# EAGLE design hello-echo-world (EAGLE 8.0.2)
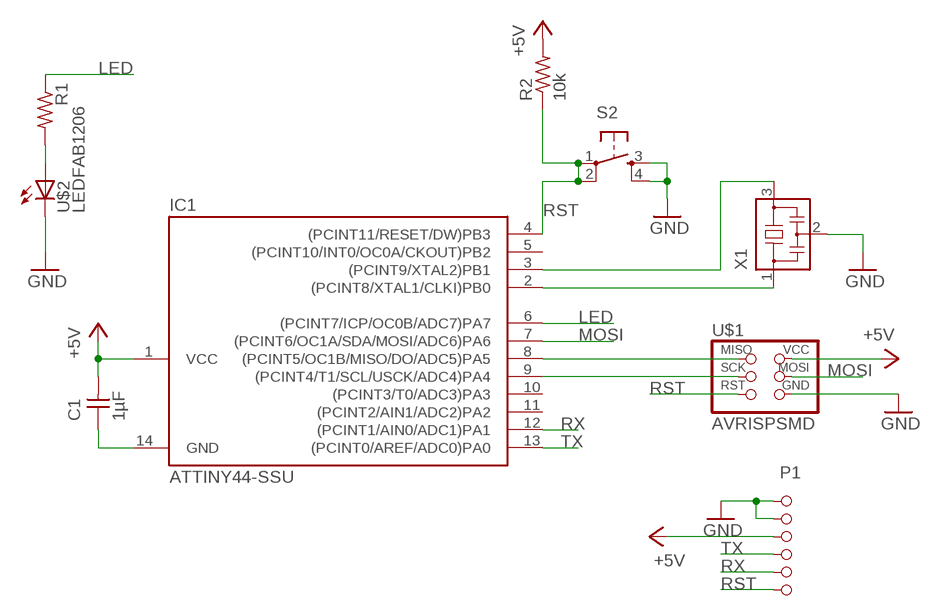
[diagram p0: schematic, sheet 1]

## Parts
C1  1µF  CAP-UNPOLARIZEDFAB  [C1206FAB]
IC1  ATTINY44-SSU  [SOIC14]
P1  SMD-6  [SMD-6]
R1  RES-US1206FAB  [R1206FAB]
R2  10k  RES-US1206FAB  [R1206FAB]
S2  6MM_SWITCH6MM_SWITCH  [6MM_SWITCH]
U$1  AVRISPSMD  [2X03SMD]
U$2  LEDFAB1206  [LED1206FAB]
X1  RESONATOR-PBRC  [PBRC]

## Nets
+5V: C1.2 IC1.1(VCC) P1.P$3 R2.2 U$1.2(VCC)
GND: C1.1 IC1.14(GND) P1.P$1 P1.P$2 S2.3(S) S2.4(S1) U$1.6(GND) U$2.2(C) X1.2
LED: IC1.6((PCINT7/ICP/OC0B/ADC7)PA7) R1.1
MOSI: IC1.7((PCINT6/OC1A/SDA/MOSI/ADC6)PA6) U$1.4(MOSI)
N$3: IC1.2((PCINT8/XTAL1/CLKI)PB0) X1.1
N$4: IC1.3((PCINT9/XTAL2)PB1) X1.3
N$5: IC1.8((PCINT5/OC1B/MISO/DO/ADC5)PA5) U$1.1(MISO)
N$6: IC1.9((PCINT4/T1/SCL/USCK/ADC4)PA4) U$1.3(SCK)
N$7: R1.2 U$2.1(A)
RST: IC1.4((PCINT11/RESET/DW)PB3) P1.P$6 R2.1 S2.1(P) S2.2(P1) U$1.5(RST)
RX: IC1.12((PCINT1/AIN0/ADC1)PA1) P1.P$5
TX: IC1.13((PCINT0/AREF/ADC0)PA0) P1.P$4
Unconnected: IC1.5((PCINT10/INT0/OC0A/CKOUT)PB2) IC1.10((PCINT3/T0/ADC3)PA3) IC1.11((PCINT2/AIN1/ADC2)PA2)

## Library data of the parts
C1 = fab:CAP-UNPOLARIZED
IC1 = fab:ATTINY44
P1 = PinHeader:SMD-6
R1 R2 = fab:RES-US: Resistor (US Symbol)
S2 = fab:6MM_SWITCH: OMRON SWITCH
U$1 = fab:AVRISP
U$2 = fab:LED: LED
X1 = fab:RESONATOR-PBRC

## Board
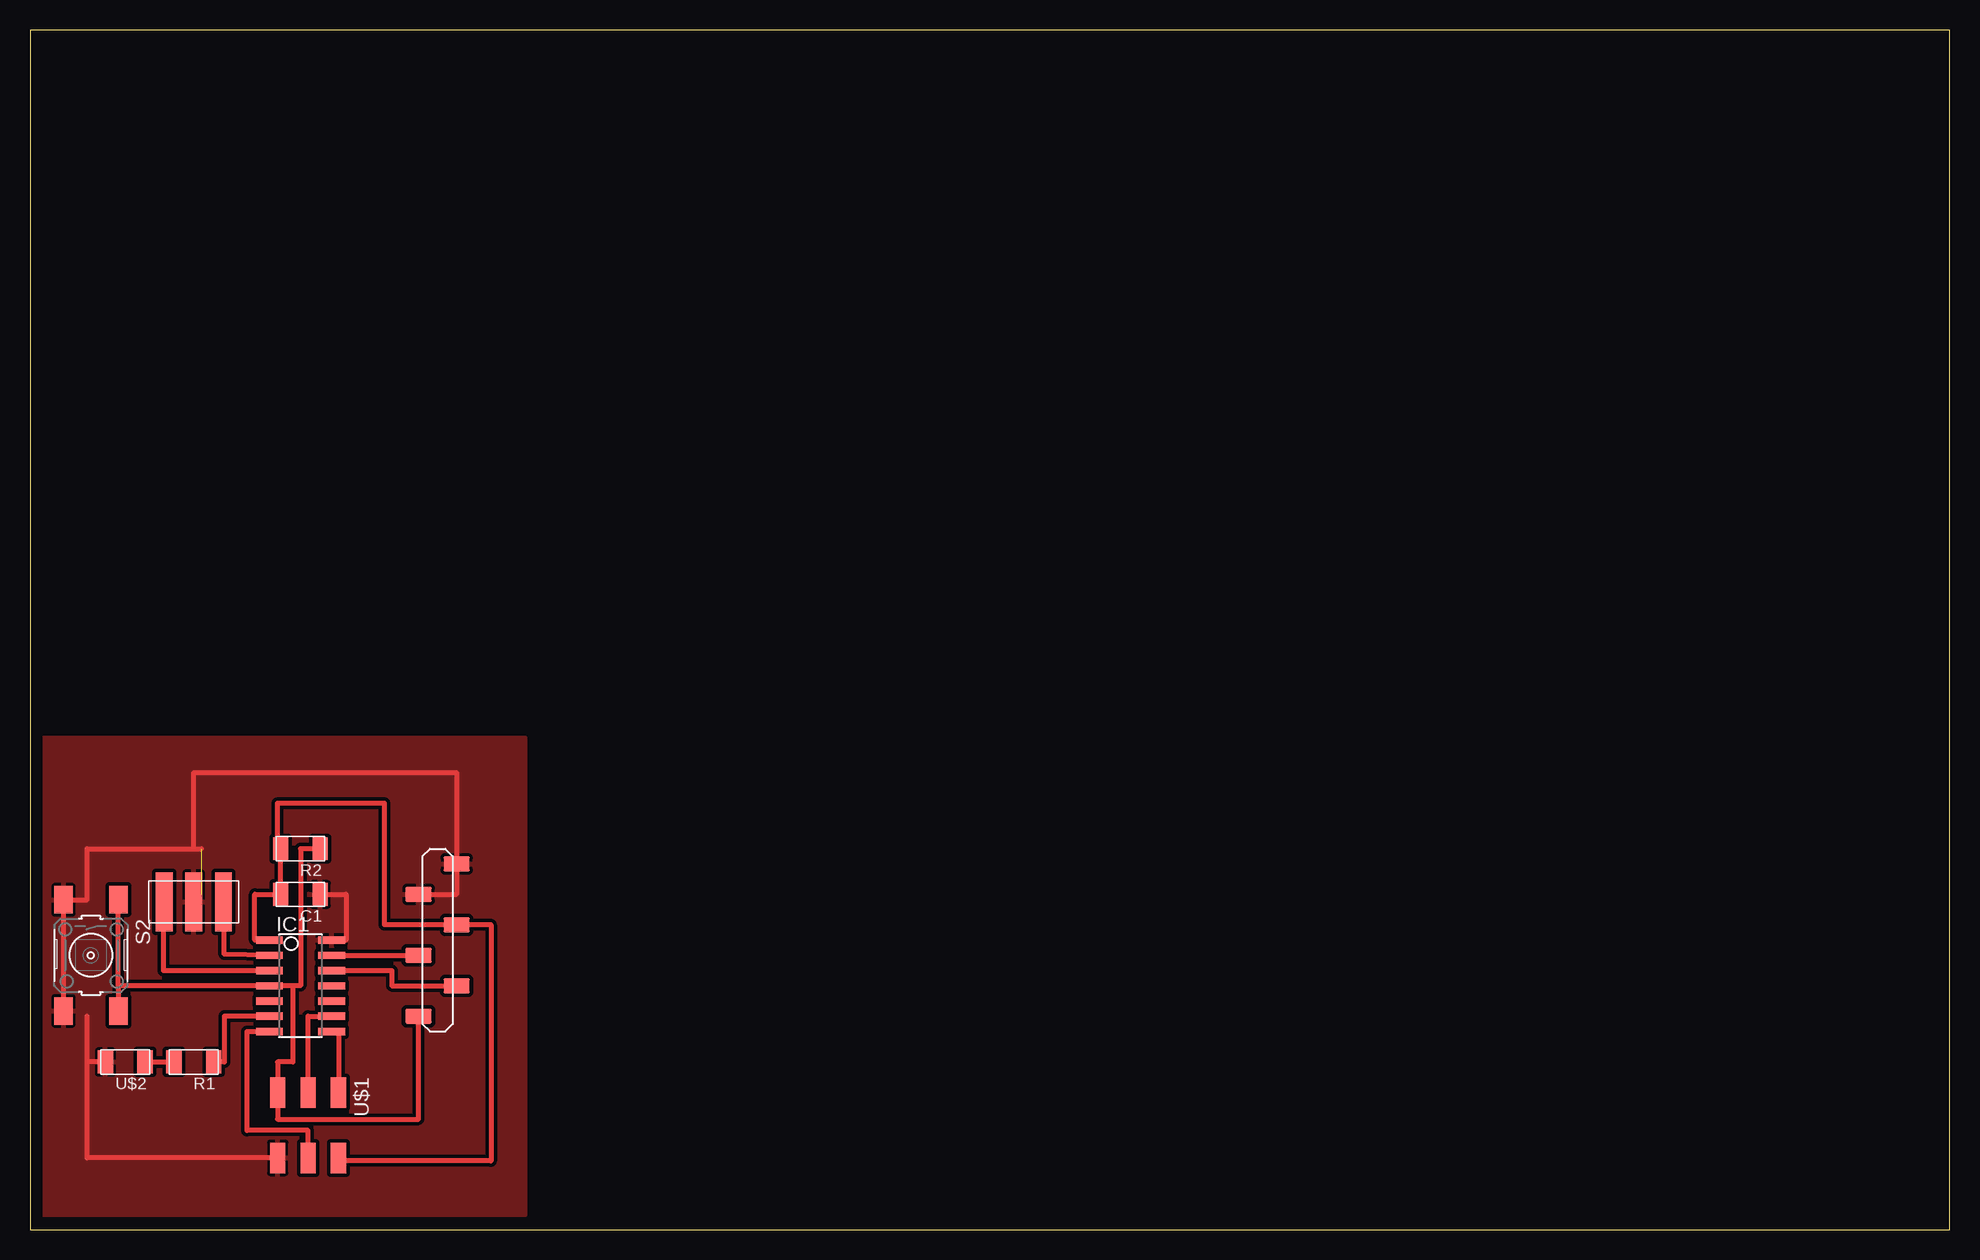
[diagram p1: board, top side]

Size 160 x 100 mm. Coordinates in mm from the lower left corner, seen from the top.
Outline: 0,0 160,0 160,100 0,100 0,0
Copper layers (1*16): Top 0.035mm / dielectric 1.5mm / Bottom 0.035mm
Design rules "default *": minimum track width 10mil, minimum drill 24mil, track to track 0.3mm, track to pad 0.3mm, pad to pad 0.3mm, via to via 8mil, smd to smd 8mil, copper to edge 40mil, drill to drill 8mil, minimum pad ring 10mil, minimum via ring 8mil, stop-mask expansion 0.3mm, vias tented up to drill 0mil, thermal gap 10mil

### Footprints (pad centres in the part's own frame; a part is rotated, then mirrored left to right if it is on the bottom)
C1206FAB = smd 1.27 x 1.905: 1 -1.651,0; 2 1.651,0
SOIC14 = smd 0.61 x 2.21: 1 -3.81,-2.603; 2 -2.54,-2.603; 3 -1.27,-2.603; 4 0,-2.603; 5 1.27,-2.603; 6 2.54,-2.603; 7 3.81,-2.603; 8 3.81,2.603; 9 2.54,2.603; 10 1.27,2.603; 11 0,2.603; 12 -1.27,2.603; 13 -2.54,2.603; 14 -3.81,2.603
SMD-6 = smd 1.27 x 2.2: P$1 -6.35,1.587; P$2 -3.81,-1.587; P$3 -1.27,1.587; P$4 1.27,-1.587; P$5 3.81,1.587; P$6 6.35,-1.587
R1206FAB = smd 1.27 x 1.905: 1 -1.651,0; 2 1.651,0
6MM_SWITCH = smd 2.286 x 1.524: 1 -4.637,2.286; 2 4.637,2.286; 3 -4.637,-2.286; 4 4.637,-2.286
2X03SMD = smd 2.54 x 1.27: 1 -2.54,2.54; 2 2.92,2.54; 3 -2.54,0; 4 2.92,0; 5 -2.54,-2.54; 6 2.92,-2.54
LED1206FAB = smd 1.27 x 1.905: 1 -1.651,0; 2 1.651,0
PBRC = smd 1.4 x 4.9: 1 -2.475,0; 2 0,0; 3 2.475,0

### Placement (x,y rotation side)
C1  22.54,27.94 180 top
IC1  22.54,20.32 270 top
P1  33.97,24.13 270 top
R1  13.65,13.97 180 top
R2  22.54,31.75 180 top
S2  5.08,22.86 270 top
U$1  23.18,8.89 270 top
U$2  7.94,13.97 180 top
X1  13.65,27.3 180 top

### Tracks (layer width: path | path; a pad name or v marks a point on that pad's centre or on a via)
+5V
  Top 0.406: U$1.2 25.72,5.71 38.42,5.71 38.42,25.4 P1.P$3 29.53,25.4 29.53,35.56 20.64,35.56 20.64,31.75 R2.2 C1.2 18.73,27.94 18.73,24.13 IC1.1
GND  (1 unrouted)
  Top 0.406: S2.4 S2.3 4.76,27.5 4.76,31.75 13.65,31.75 | U$2.2 4.76,13.97 | P1.P$2 35.56,27.94 P1.P$1 35.56,38.1 13.65,38.1 13.65,31.75 | 4.76,13.97 4.76,5.97 U$1.6 | 4.76,13.97 4.76,17.78 | 13.65,31.75 14.29,31.75 | C1.1 26.35,27.94 26.35,24.13
  pour Top (isolate 0.305): 0.95,40.96 0.95,1.27 41.27,1.27 41.27,40.96
LED
  Top 0.406: IC1.6 16.19,17.78 16.19,13.97 R1.1
MOSI
  Top 0.406: IC1.7 18.1,16.51 18.1,8.26 23.18,8.26 U$1.4
N$3
  Top 0.406: 19.94,22.94 IC1.2 16.19,22.94 X1.1
N$4
  Top 0.406: X1.3 11.11,24.13 11.11,21.59 IC1.3
N$5
  Top 0.406: IC1.8 25.72,16.51 U$1.1
N$6
  Top 0.406: U$1.3 23.18,17.78 IC1.9
N$7
  Top 0.406: U$2.1 R1.2
RST
  Top 0.406: 7.37,20.32 S2.2 | 7.37,20.32 S2.1 | R2.1 22.54,31.75 22.54,20.32 21.91,20.32 | 21.91,20.32 IC1.4 7.37,20.32 | 21.91,20.32 21.91,13.97 20.64,13.97 U$1.5 20.64,9.21 32.38,9.21 P1.P$6
RX
  Top 0.406: IC1.12 30.16,21.59 30.16,20.32 P1.P$5
TX
  Top 0.406: IC1.13 P1.P$4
